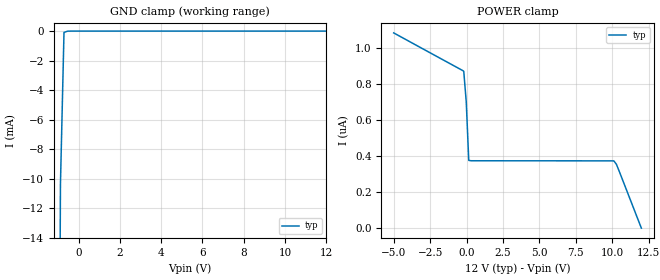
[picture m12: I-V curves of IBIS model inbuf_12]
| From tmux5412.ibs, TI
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| inbuf_12
[Model]   inbuf_12
Model_type   Input
Vinl = 0.8
Vinh = 1.3
|   typ   min   max
C_comp   1.598234e-12   NA   NA
[Voltage Range]   12   NA   NA
[Temperature Range]   27   NA   NA
[Power Clamp Reference]   12   NA   NA
[GND Clamp Reference]   0   NA   NA
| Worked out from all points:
|   GND clamp passes 1 mA (typ) near -0.72 V on its own axis
[GND Clamp]
|   Voltage   I(typ)   I(min)   I(max)
-5V       -4.814A    NA         NA
-1.051V   -59.57mA   NA         NA
-878.8mV  -10.37mA   NA         NA
-707.1mV  -90.71uA   NA         NA
-535.4mV  -4.868uA   NA         NA
-363.6mV  -107.9nA   NA         NA
12V       616.9nA    NA         NA
[POWER Clamp]
|   Voltage   I(typ)   I(min)   I(max)
-5V       1.086uA    NA         NA
-191.9mV  872.7nA    NA         NA
-20.2mV   702.1nA    NA         NA
151.5mV   376.9nA    NA         NA
10.11V    373.9nA    NA         NA
10.28V    355.9nA    NA         NA
12V       -62.03pA   NA         NA
